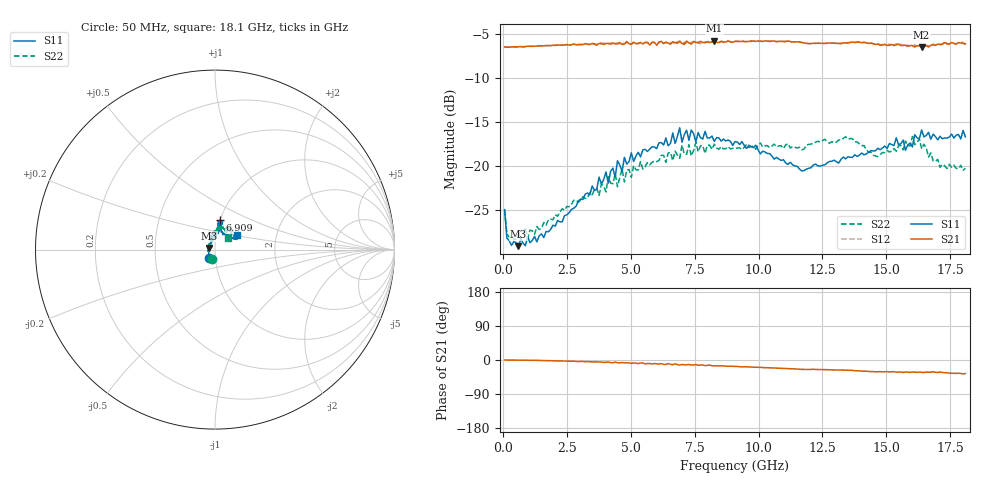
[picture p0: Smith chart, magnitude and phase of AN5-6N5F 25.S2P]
! Network Analyzer HP8720D.06.14 Serial No. US36140669
!  6 Jul 2005  08:05:57
! Frequency  S11  S21  S12  S22
# HZ  S  DB R 50
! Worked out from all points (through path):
!   201 points, 50 MHz to 18.1 GHz, reference 50 ohm
!   highest |S21| = -5.79 dB at 8.263 GHz (marker M1); lowest = -6.5 dB at 16.39 GHz (marker M2)
!   group delay of S21, straight-line fit = 5.97 ps
!   lowest |S11| = -29.1 dB at 591.5 MHz (marker M3), VSWR 1.07, Z = 46.7 + j0.833 ohm
!   |S11| at or under -10 dB: start of sweep to end of sweep
!   |S22| runs from -28.3 to -16.6 dB; largest |S21 - S12| = 0.02
!   S11 on the Smith chart (normalised r, x): 50 MHz: 0.93, -0.09; 6.909 GHz: 1.00, +0.33; 18.1 GHz: 1.25, +0.21
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5e7  -24.92 -124.6  -6.50 0.0  -6.50 0.1  -24.98 -107.5
1.4025e8  -28.15 -152.5  -6.54 -0.0  -6.52 -0.1  -27.64 -151.8
5.915e8  -29.05 165.4  -6.48 -0.3  -6.49 -0.2  -27.58 169.2
3.1185e9  -23.76 95.9  -6.23 -3.9  -6.25 -4.2  -23.45 111.2
4.021e9  -20.66 87.6  -6.11 -6.2  -6.19 -5.5  -22.91 100.6
4.382e9  -21.24 83.6  -6.16 -5.8  -6.12 -7.1  -20.85 100.0
4.47225e9  -19.38 79.2  -6.15 -7.2  -6.06 -6.2  -22.33 102.5
4.65275e9  -20.58 78.8  -6.23 -6.6  -6.05 -7.5  -20.32 100.8
4.743e9  -19.00 82.2  -6.17 -7.6  -6.15 -6.8  -21.79 96.4
6.09675e9  -17.36 78.2  -5.97 -10.5  -5.91 -10.4  -19.36 85.7
6.7285e9  -17.42 83.1  -6.01 -10.1  -6.21 -11.1  -18.29 79.3
6.909e9  -15.66 80.9  -5.84 -13.3  -5.97 -11.9  -19.10 77.0
6.99925e9  -17.28 80.3  -6.12 -11.7  -6.20 -13.3  -17.64 78.7
7.36025e9  -15.91 74.2  -6.18 -13.4  -5.98 -12.4  -18.84 82.3
7.54075e9  -17.24 75.6  -5.98 -12.1  -5.86 -14.3  -17.30 80.8
8.26275e9  -17.20 81.0  -5.79 -15.5  -5.94 -16.0  -17.50 69.9
9.075e9  -17.21 79.4  -5.88 -16.9  -5.86 -16.9  -17.93 68.1
1.21435e10  -19.86 59.7  -6.09 -24.6  -6.05 -24.7  -17.44 63.9
1.512175e10  -17.43 27.9  -6.32 -31.5  -6.18 -31.1  -18.40 59.7
1.57535e10  -18.21 31.0  -6.29 -31.8  -6.50 -32.7  -17.15 54.6
1.638525e10  -15.90 34.3  -6.55 -32.6  -6.34 -32.0  -18.03 45.3
1.81e10  -16.68 34.9  -6.14 -35.9  -6.26 -36.4  -20.24 41.7
